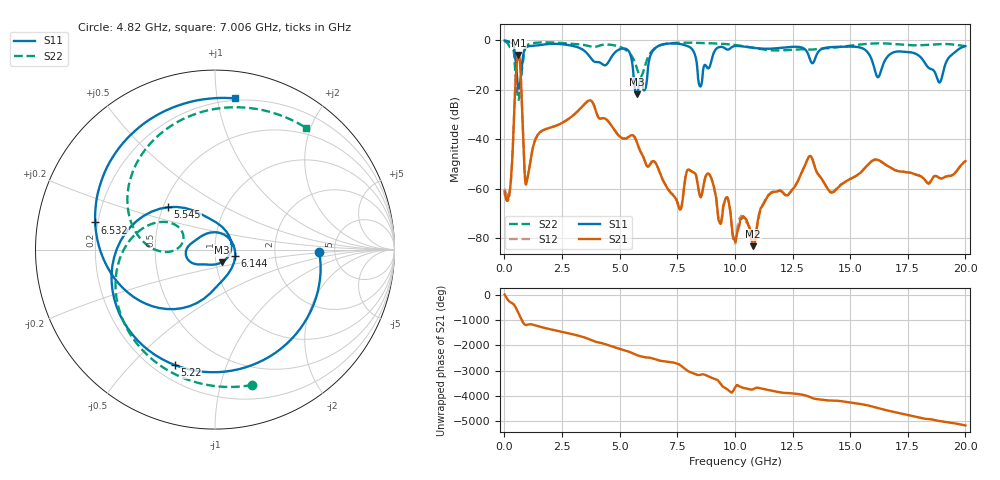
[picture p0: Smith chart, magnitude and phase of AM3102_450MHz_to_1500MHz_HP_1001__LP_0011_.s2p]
!Agilent Technologies,E8364B,MY43040894,A.07.50.67
!Agilent E8364B: A.07.50.67
!Date: Thursday, January 11, 2018 06:01:39
!Correction: S11(Full 2 Port(1,2))
!S21(Full 2 Port(1,2))
!S12(Full 2 Port(1,2))
!S22(Full 2 Port(1,2))
!S2P File: Measurements: S11, S21, S12, S22:
# Hz S  dB  R 50
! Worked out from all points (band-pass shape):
!   1601 points, 10 MHz to 20 GHz, reference 50 ohm
!   highest |S21| = -5.97 dB at 609.7 MHz (marker M1); lowest = -83.3 dB at 10.79 GHz (marker M2)
!   |S21| within 3 dB of the highest: 544.4 MHz to 677 MHz (132.6 MHz wide, 21.7 % of centre)
!   lowest |S11| = -21.9 dB at 5.745 GHz (marker M3), VSWR 1.17, Z = 53.6 - j7.53 ohm
!   |S11| at or under -10 dB: 5.559 GHz to 6.245 GHz (686.3 MHz wide, 11.6 % of centre); 16.01 GHz to 16.42 GHz (410.7 MHz wide, 2.53 % of centre); 18.3 GHz to 19.12 GHz (817.2 MHz wide, 4.37 % of centre)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
!   |S22| runs from -24.1 to -0.4 dB; largest |S21 - S12| = 0.00072
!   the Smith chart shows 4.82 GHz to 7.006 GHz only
!   S11 on the Smith chart (normalised r, x): 4.82 GHz: 3.77, -0.14; 5.22 GHz: 0.28, -0.67; 5.545 GHz: 0.53, +0.29; 6.144 GHz: 1.25, -0.09; 6.532 GHz: 0.19, +0.11; 7.006 GHz: 0.19, +1.13
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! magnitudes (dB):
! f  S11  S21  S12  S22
! 10 MHz  -0.1  -61.2  -60.1  -0.4
! 247.4 MHz  -0.8  -60.2  -60.1  -2.8
! 609.7 MHz  -19.3  -6.0  -6.0  -24.0
! 972 MHz  -2.7  -57.1  -57.0  -2.2
! 1.484 GHz  -2.0  -37.8  -37.8  -0.9
! 3.346 GHz  -3.5  -27.1  -27.1  -1.7
! 4.82 GHz  -4.7  -36.9  -36.9  -2.1
! 5.22 GHz  -3.3  -39.8  -39.8  -3.6
! 5.545 GHz  -9.0  -38.4  -38.4  -6.7
! 5.745 GHz  -21.9  -41.1  -41.1  -11.1
! 6.144 GHz  -18.5  -50.2  -50.2  -8.9
! 6.532 GHz  -3.3  -49.3  -49.3  -3.2
! 6.682 GHz  -2.3  -52.1  -52.1  -2.4
! 7.006 GHz  -1.4  -58.8  -58.7  -1.4
! 8.868 GHz  -11.3  -54.0  -54.0  -1.2
! 10.01 GHz  -2.3  -81.4  -82.1  -1.9
! 10.79 GHz  -3.0  -83.3  -81.2  -3.1
! 13.34 GHz  -9.2  -47.6  -47.6  -3.8
! 14.2 GHz  -2.7  -61.7  -61.4  -3.1
! 16.68 GHz  -6.1  -51.1  -51.1  -1.3
! 18.88 GHz  -17.1  -55.8  -55.7  -1.5
! 20 GHz  -2.4  -48.9  -49.0  -2.3
